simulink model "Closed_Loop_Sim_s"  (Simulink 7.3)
settings: Solver=ode4  StartTime=0.0  StopTime=100  FixedStep=0.002  RelTol=1e-3
InitFcn:
  | d2r=pi/180; r2d=180/pi;
  | [Av1, Bv1, Cv1, Dv1]= plant_flxcont;              % Continuous Plant
  | [Acs, Bcs, Ccs, Dcs]= controller_s;               % Continuous Stage-2 Controller
StartFcn:
  | d2r=pi/180; r2d=180/pi;
  | [Av1, Bv1, Cv1, Dv1]= plant_flxcont;              % Continuous Plant
  | [Acs, Bcs, Ccs, Dcs]= controller_s;               % Continuous Stage-2 Controller
StopFcn:
  | Pl
undefined symbols (not defined in the file or in its folder): Acs, Av1, Bcs, Bv1, Ccs, Coulomb_Damper, Cv1, Dcs, Dv1

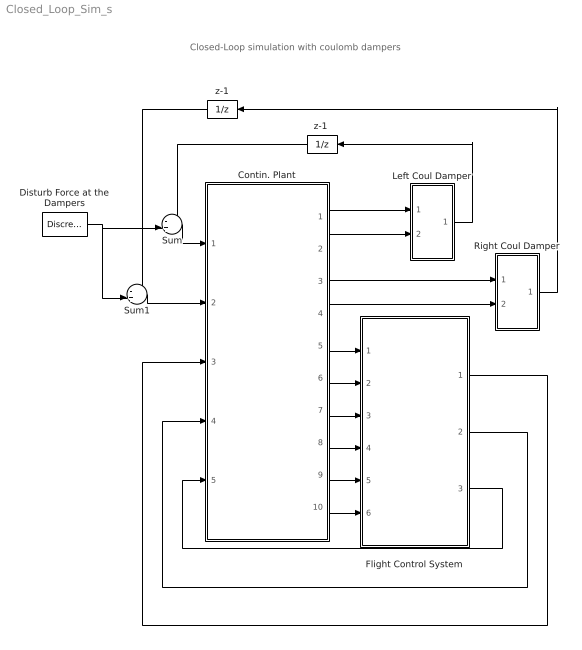
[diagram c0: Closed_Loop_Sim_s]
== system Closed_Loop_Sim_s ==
  note: Closed-Loop simulation with coulomb dampers
  Contin. Plant : Subsystem
  Disturb Force at the Dampers : DiscretePulseGenerator  PulseType=Time based  Amplitude=175  Period=800  PulseWidth=0.2  PhaseDelay=0  SampleTime=1
  Flight Control System : Subsystem
  Left Coul Damper : Subsystem
  Right Coul Damper : Subsystem
  Sum : Sum  Inputs=-+|  OutDataType=sfix(16)  OutScaling=2^0
  Sum1 : Sum  Inputs=-+|  OutDataType=sfix(16)  OutScaling=2^0
  z-1 : UnitDelay  SampleTime=0.002
  "z-1 " : UnitDelay  SampleTime=0.002
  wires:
  Sum/1 -> Contin. Plant/1(F-left)
  Sum1/1 -> Contin. Plant/2(F-right)
  Disturb Force at the Dampers/1 -> Sum/2, Sum1/2
  Left Coul Damper/1(Fcd) -> "z-1 "/1
  Right Coul Damper/1(Fcd) -> z-1/1
  Contin. Plant/1(dZ-Left) -> Left Coul Damper/1(Ext)
  Contin. Plant/2(dZ-dot-Left) -> Left Coul Damper/2(Rate)
  "z-1 "/1 -> Sum/1
  z-1/1 -> Sum1/1
  Contin. Plant/5(phi) -> Flight Control System/1(Phi)
  Contin. Plant/6(theta) -> Flight Control System/2(Theta)
  Contin. Plant/7(psi) -> Flight Control System/3(Psi)
  Contin. Plant/8(P) -> Flight Control System/4(P)
  Contin. Plant/9(Q) -> Flight Control System/5(Q)
  Contin. Plant/10(R) -> Flight Control System/6(R)
  Flight Control System/1(DP-TVC) -> Contin. Plant/3(DP)
  Flight Control System/2(DQ-TVC) -> Contin. Plant/4(DQ)
  Flight Control System/3(DR-TVC) -> Contin. Plant/5(DR)
  Contin. Plant/3(dZ-Rght) -> Right Coul Damper/1(Ext)
  Contin. Plant/4(dZ-dot-Rght) -> Right Coul Damper/2(Rate)

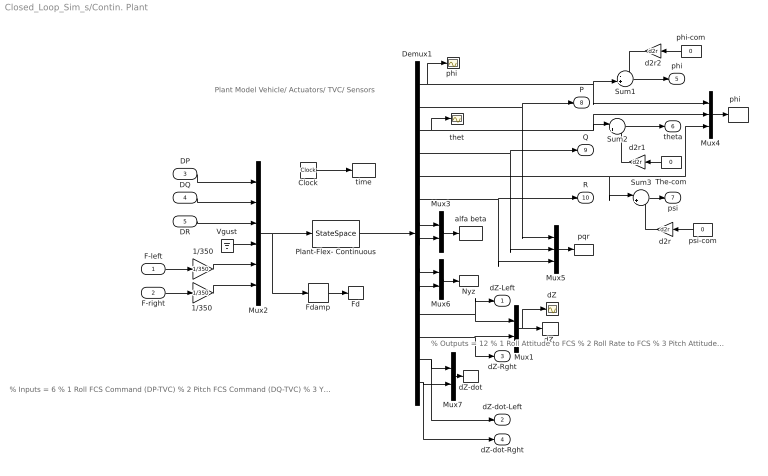
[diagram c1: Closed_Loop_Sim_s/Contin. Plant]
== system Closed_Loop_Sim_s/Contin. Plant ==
  note: Plant Model Vehicle/ Actuators/ TVC/ Sensors
  note: % Inputs = 6 % 1 Roll FCS Command (DP-TVC) % 2 Pitch FCS Command (DQ-TVC) % 3 Yaw FCS Command (DR-TVC) % 4 Wind-Gust Velocity (ft/sec) % 5 Left Coulomb Damper Force % 6 Right Coulomb Damper Force
  note: % Outputs = 12 % 1 Roll Attitude to FCS % 2 Roll Rate to FCS % 3 Pitch Attitude to FCS % 4 Pitch Rate to FCS % 5 Yaw Attitude to FCS % 6 Yaw Rate to FCS % 7 Angle of Attack, alpha (rad) % 8 Angle of Sideslip, beta (rad) % 9 Normal Accelerometer, Nz (ft/sec^2) % 10 Lateral Accelerometer, Ny (ft/sec^2) % 11 Left Damper Extension (ft) % 12 Right Damper Extension (ft) % 13 Left Damper Rate (ft/sec) % 14 Right Damper Rate (ft/s)
  F-left : Inport  OutDataType=sfix(16)  OutScaling=2^0
  F-right : Inport  Port=2  OutDataType=sfix(16)  OutScaling=2^0
  DP : Inport  Port=3  OutDataType=sfix(16)  OutScaling=2^0
  DQ : Inport  Port=4  OutDataType=sfix(16)  OutScaling=2^0
  DR : Inport  Port=5  OutDataType=sfix(16)  OutScaling=2^0
  1/350 : Gain  Gain=1/350  ParameterDataType=fixdt(1, 16)  ParameterScaling=2^0  OutDataType=fixdt(1, 16)  OutScaling=2^0
  "1/350 " : Gain  Gain=1/350  ParameterDataType=fixdt(1, 16)  ParameterScaling=2^0  OutDataType=fixdt(1, 16)  OutScaling=2^0
  Clock : Clock
  Demux1 : Demux  Outputs=14
  Fd : ToWorkspace  VariableName=Fd  SampleTime=-1  SaveFormat=Array
  Fdamp : Selector  InputPortWidth=6  IndexOptions=Index vector (dialog)  Indices="[5  6]"  OutputSizes=1
  Mux{1,3,6..7} (4 alike) : Mux  Inputs=2
  Mux2 : Mux  Inputs=6
  Mux4 : Mux  Inputs=3
  Mux5 : Mux  Inputs=3
  Nyz : ToWorkspace  VariableName=Nyz  SampleTime=-1  SaveFormat=Array
  Plant-Flex- Continuous : StateSpace  A=Av1  B=Bv1  C=Cv1  D=Dv1
  Sum1 : Sum  Inputs=-+|  OutDataType=sfix(16)  OutScaling=2^0
  Sum2 : Sum  Inputs=|+-  OutDataType=sfix(16)  OutScaling=2^0
  Sum3 : Sum  Inputs=|+-  OutDataType=sfix(16)  OutScaling=2^0
  The-com : Constant  Value=0  OutDataType=sfix(16)  OutScaling=2^0
  Vgust : Ground
  alfa beta : ToWorkspace  VariableName=albet  SampleTime=-1  SaveFormat=Array
  d2r : Gain  Gain=d2r  ParameterDataType=sfix(16)  ParameterScaling=2^0  OutDataType=sfix(16)  OutScaling=2^0
  d2r1 : Gain  Gain=d2r  ParameterDataType=sfix(16)  ParameterScaling=2^0  OutDataType=sfix(16)  OutScaling=2^0
  d2r2 : Gain  Gain=d2r  ParameterDataType=sfix(16)  ParameterScaling=2^0  OutDataType=sfix(16)  OutScaling=2^0
  dZ : Scope
  "dZ " : ToWorkspace  VariableName=dZ  SampleTime=-1  SaveFormat=Array
  dZ-dot : ToWorkspace  VariableName=dZd  SampleTime=-1  SaveFormat=Array
  "phi " : Scope
  "phi   " : ToWorkspace  VariableName=attit  SampleTime=-1  SaveFormat=Array
  phi-com : Constant  Value=0  OutDataType=sfix(16)  OutScaling=2^0
  pqr : ToWorkspace  VariableName=pqr  SampleTime=-1  SaveFormat=Array
  psi-com : Constant  Value=0  OutDataType=sfix(16)  OutScaling=2^0
  thet : Scope
  time : ToWorkspace  VariableName=time  SampleTime=-1  SaveFormat=Array
  dZ-Left : Outport  OutDataType=sfix(16)  OutScaling=2^0
  dZ-dot-Left : Outport  Port=2  OutDataType=sfix(16)  OutScaling=2^0
  dZ-Rght : Outport  Port=3  OutDataType=sfix(16)  OutScaling=2^0
  dZ-dot-Rght : Outport  Port=4  OutDataType=sfix(16)  OutScaling=2^0
  phi : Outport  Port=5  OutDataType=sfix(16)  OutScaling=2^0
  theta : Outport  Port=6  OutDataType=sfix(16)  OutScaling=2^0
  psi : Outport  Port=7  OutDataType=sfix(16)  OutScaling=2^0
  P : Outport  Port=8  OutDataType=sfix(16)  OutScaling=2^0
  Q : Outport  Port=9  OutDataType=sfix(16)  OutScaling=2^0
  R : Outport  Port=10  OutDataType=sfix(16)  OutScaling=2^0
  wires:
  F-left/1 -> 1/350/1
  F-right/1 -> "1/350 "/1
  DP/1 -> Mux2/1
  DQ/1 -> Mux2/2
  DR/1 -> Mux2/3
  Demux1/7 -> Mux3/1
  Demux1/9 -> Mux6/1
  Demux1/11 -> dZ-Left/1, Mux1/1
  Demux1/12 -> dZ-Rght/1, Mux1/2
  Mux2/1 -> Plant-Flex- Continuous/1, Fdamp/1
  Mux3/1 -> alfa beta/1
  Mux6/1 -> Nyz/1
  Vgust/1 -> Mux2/4
  Demux1/6 -> R/1, Mux5/3
  Plant-Flex- Continuous/1 -> Demux1/1
  Demux1/13 -> Mux7/1, dZ-dot-Left/1
  Demux1/14 -> Mux7/2, dZ-dot-Rght/1
  Sum2/1 -> theta/1
  Demux1/3 -> Sum2/1, Mux4/2, thet/1
  The-com/1 -> d2r1/1
  Demux1/1 -> "phi "/1, Sum1/2, Mux4/1
  Sum1/1 -> phi/1
  phi-com/1 -> d2r2/1
  Sum3/1 -> psi/1
  Demux1/5 -> Mux4/3, Sum3/1
  psi-com/1 -> d2r/1
  Demux1/4 -> Q/1, Mux5/2
  Mux4/1 -> "phi   "/1
  Mux1/1 -> "dZ "/1, dZ/1
  Fdamp/1 -> Fd/1
  Clock/1 -> time/1
  Mux5/1 -> pqr/1
  Demux1/2 -> P/1, Mux5/1
  Mux7/1 -> dZ-dot/1
  d2r2/1 -> Sum1/1
  d2r1/1 -> Sum2/2
  d2r/1 -> Sum3/2
  Demux1/8 -> Mux3/2
  Demux1/10 -> Mux6/2
  "1/350 "/1 -> Mux2/6
  1/350/1 -> Mux2/5

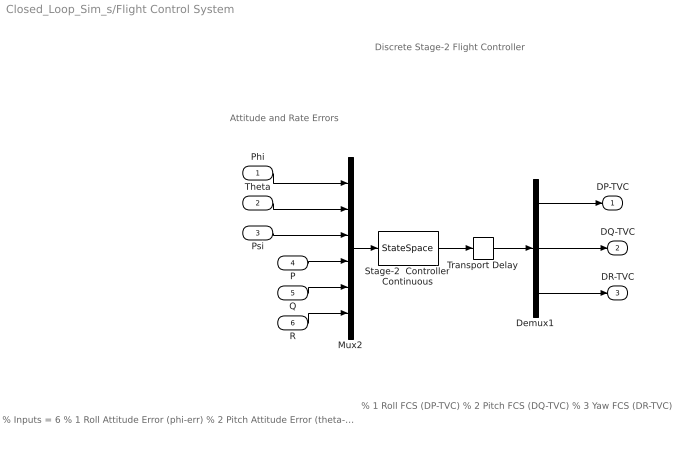
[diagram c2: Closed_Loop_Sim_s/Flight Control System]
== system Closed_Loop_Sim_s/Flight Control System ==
  note: Discrete Stage-2 Flight Controller
  note: Attitude and Rate Errors
  note: % Inputs = 6 % 1 Roll Attitude Error (phi-err) % 2 Pitch Attitude Error (theta-err) % 3 Yaw Attitude Error (psi-err) % 4 Roll Rate Error (p-err) % 5 Pitch Rate Error (q-err) % 6 Yaw Rate Error (r-err)
  note: % 1 Roll FCS (DP-TVC) % 2 Pitch FCS (DQ-TVC) % 3 Yaw FCS (DR-TVC)
  Phi : Inport  OutDataType=sfix(16)  OutScaling=2^0
  Theta : Inport  Port=2  OutDataType=sfix(16)  OutScaling=2^0
  Psi : Inport  Port=3  OutDataType=sfix(16)  OutScaling=2^0
  P : Inport  Port=4  OutDataType=sfix(16)  OutScaling=2^0
  Q : Inport  Port=5  OutDataType=sfix(16)  OutScaling=2^0
  R : Inport  Port=6  OutDataType=sfix(16)  OutScaling=2^0
  Demux1 : Demux  Outputs=3
  Mux2 : Mux  Inputs=6
  Stage-2  Controller Continuous : StateSpace  A=Acs  B=Bcs  C=Ccs  D=Dcs
  Transport Delay : TransportDelay  DelayTime=0.04  PadeOrder=2
  DP-TVC : Outport  OutDataType=sfix(16)  OutScaling=2^0
  DQ-TVC : Outport  Port=2  OutDataType=sfix(16)  OutScaling=2^0
  DR-TVC : Outport  Port=3  OutDataType=sfix(16)  OutScaling=2^0
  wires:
  Q/1 -> Mux2/5
  R/1 -> Mux2/6
  Phi/1 -> Mux2/1
  Theta/1 -> Mux2/2
  Psi/1 -> Mux2/3
  Mux2/1 -> Stage-2  Controller Continuous/1
  Stage-2  Controller Continuous/1 -> Transport Delay/1
  P/1 -> Mux2/4
  Demux1/2 -> DQ-TVC/1
  Demux1/1 -> DP-TVC/1
  Demux1/3 -> DR-TVC/1
  Transport Delay/1 -> Demux1/1

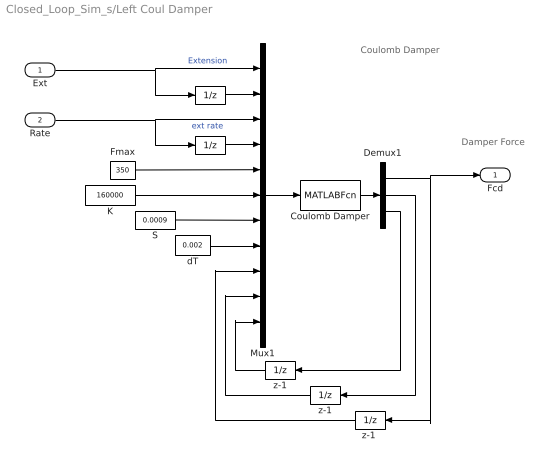
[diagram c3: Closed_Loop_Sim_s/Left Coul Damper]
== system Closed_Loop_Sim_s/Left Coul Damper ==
  note: Coulomb Damper
  note: Damper Force
  Ext : Inport  OutDataType=sfix(16)  OutScaling=2^0
  Rate : Inport  Port=2  OutDataType=sfix(16)  OutScaling=2^0
  " " : UnitDelay  SampleTime=0.002
  "   " : UnitDelay  SampleTime=0.002
  " z-1 " : UnitDelay  SampleTime=0.002
  Coulomb Damper : MATLABFcn  MATLABFcn=Coulomb_Damper(u(1),u(2),u(3),u(4), u(5),u(6),u(7),u(8), u(9),u(10),u(11) )  OutputDimensions=3  SampleTime=0.002
  Demux1 : Demux  Outputs=3
  Fmax : Constant  Value=350  OutDataType=sfix(16)  OutScaling=2^0
  K : Constant  Value=160000  OutDataType=sfix(16)  OutScaling=2^0
  Mux1 : Mux  Inputs=11
  S : Constant  Value=0.0009  OutDataType=sfix(16)  OutScaling=2^0
  dT : Constant  Value=0.002  OutDataType=sfix(16)  OutScaling=2^0
  z-1 : UnitDelay  SampleTime=0.002
  "z-1 " : UnitDelay  SampleTime=0.002
  Fcd : Outport  OutDataType=sfix(16)  OutScaling=2^0
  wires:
  Coulomb Damper/1 -> Demux1/1
  Demux1/3 -> z-1/1
  Demux1/2 -> " z-1 "/1
  Demux1/1 -> "z-1 "/1, Fcd/1
  z-1/1 -> Mux1/11
  " z-1 "/1 -> Mux1/10
  "z-1 "/1 -> Mux1/9
  Ext/1 -> " "/1, Mux1/1  "Extension"
  " "/1 -> Mux1/2
  "   "/1 -> Mux1/4
  Rate/1 -> "   "/1, Mux1/3  "ext rate"
  Fmax/1 -> Mux1/5
  K/1 -> Mux1/6
  S/1 -> Mux1/7
  Mux1/1 -> Coulomb Damper/1
  dT/1 -> Mux1/8

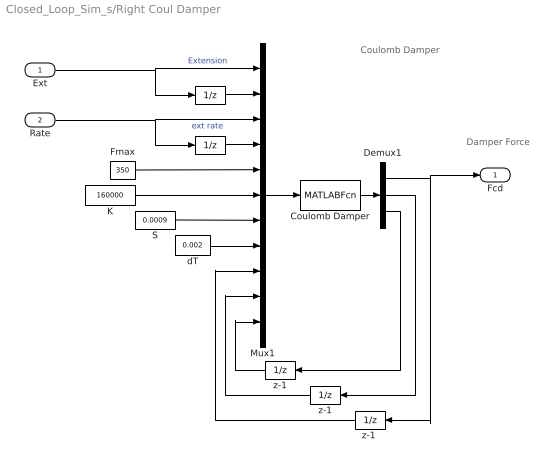
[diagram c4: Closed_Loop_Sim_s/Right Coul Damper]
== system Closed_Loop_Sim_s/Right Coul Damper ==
  note: Coulomb Damper
  note: Damper Force
  Ext : Inport  OutDataType=sfix(16)  OutScaling=2^0
  Rate : Inport  Port=2  OutDataType=sfix(16)  OutScaling=2^0
  " " : UnitDelay  SampleTime=0.002
  "   " : UnitDelay  SampleTime=0.002
  " z-1 " : UnitDelay  SampleTime=0.002
  Coulomb Damper : MATLABFcn  MATLABFcn=Coulomb_Damper(u(1),u(2),u(3),u(4), u(5),u(6),u(7),u(8), u(9),u(10),u(11) )  OutputDimensions=3  SampleTime=0.002
  Demux1 : Demux  Outputs=3
  Fmax : Constant  Value=350  OutDataType=sfix(16)  OutScaling=2^0
  K : Constant  Value=160000  OutDataType=sfix(16)  OutScaling=2^0
  Mux1 : Mux  Inputs=11
  S : Constant  Value=0.0009  OutDataType=sfix(16)  OutScaling=2^0
  dT : Constant  Value=0.002  OutDataType=sfix(16)  OutScaling=2^0
  z-1 : UnitDelay  SampleTime=0.002
  "z-1 " : UnitDelay  SampleTime=0.002
  Fcd : Outport  OutDataType=sfix(16)  OutScaling=2^0
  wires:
  Coulomb Damper/1 -> Demux1/1
  Demux1/3 -> z-1/1
  Demux1/2 -> " z-1 "/1
  Demux1/1 -> "z-1 "/1, Fcd/1
  z-1/1 -> Mux1/11
  " z-1 "/1 -> Mux1/10
  "z-1 "/1 -> Mux1/9
  Ext/1 -> " "/1, Mux1/1  "Extension"
  " "/1 -> Mux1/2
  "   "/1 -> Mux1/4
  Rate/1 -> "   "/1, Mux1/3  "ext rate"
  Fmax/1 -> Mux1/5
  K/1 -> Mux1/6
  S/1 -> Mux1/7
  Mux1/1 -> Coulomb Damper/1
  dT/1 -> Mux1/8
